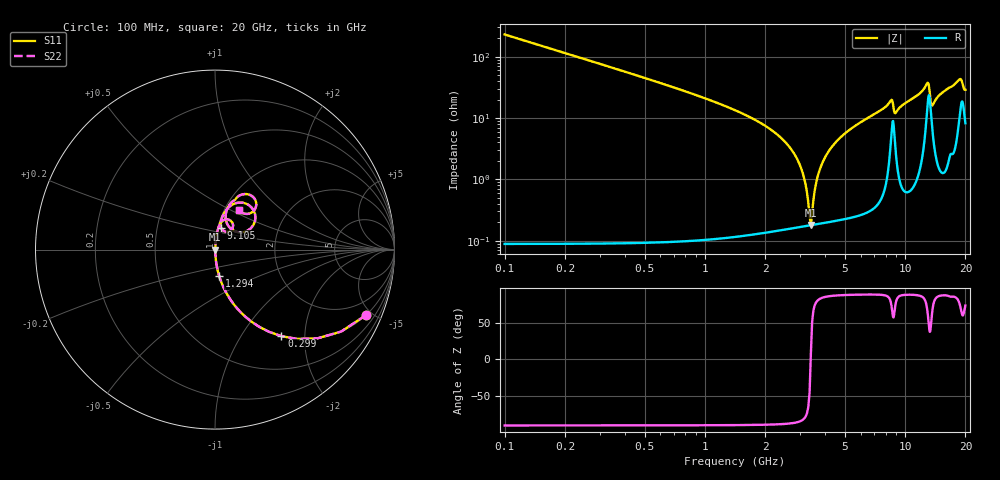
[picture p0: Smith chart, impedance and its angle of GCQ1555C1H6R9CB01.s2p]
!Murata Part Number: GCQ1555C1H6R9CB01
!These Parameters are Measured in Series Mode Connection
!Data Generated on Mar 13, 2026
!  o--ll--o
!Port1  Port2
!  o------o
!Operation Temp=25[degC], DC Bias Voltage=0[V]
!Freq. Start=100[MHz] Stop=20[GHz] 401[Steps]
# Hz S RI R 50
!Freq.(Hz) S11(Real) S11(Imag) S21(Real) S21(Imag) S12(Real) S12(Imag) S22(Real) S22(Imag)
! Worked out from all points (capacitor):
!   401 points, 100 MHz to 20 GHz, reference 50 ohm
!   read as one part in series: C = 6.9 pF near 199.5 MHz
!   lowest |Z| = 181 mohm at 3.384 GHz (marker M1)
!   series resonance near 3.378 GHz, so ESL is about 320 pH
!   S11 on the Smith chart (normalised r, x): 100 MHz: 1.00, -4.61; 299 MHz: 1.00, -1.53; 1.294 GHz: 1.00, -0.30; 9.105 GHz: 1.04, +0.26; 20 GHz: 1.16, +0.55
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1e8  0.8415 -0.3651  0.1585 0.3651  0.1585 0.3651  0.8415 -0.3651
2.99e8  0.3695 -0.4821  0.6305 0.4821  0.6305 0.4821  0.3695 -0.4821
5.975e8  0.1233 -0.3275  0.8767 0.3275  0.8767 0.3275  0.1233 -0.3275
1.294e9  0.0236 -0.1483  0.9764 0.1483  0.9764 0.1483  0.0236 -0.1483
2.7865e9  0.0023 -0.0264  0.9977 0.0264  0.9977 0.0264  0.0023 -0.0264
3.085e9  0.00185 -0.0124  0.9981 0.0124  0.9981 0.0124  0.00185 -0.0124
3.284e9  0.00177 -0.00384  0.9982 0.00384  0.9982 0.00384  0.00177 -0.00384
3.3835e9  0.00179 0.000238  0.9982 -0.000238  0.9982 -0.000238  0.00179 0.000238
3.43325e9  0.00181 0.00223  0.9982 -0.00223  0.9982 -0.00223  0.00181 0.00223
3.73175e9  0.00207 0.0137  0.9979 -0.0137  0.9979 -0.0137  0.00207 0.0137
4.279e9  0.00311 0.0327  0.9969 -0.0327  0.9969 -0.0327  0.00311 0.0327
6.7665e9  0.0145 0.1061  0.9855 -0.1061  0.9855 -0.1061  0.0145 0.1061
8.50775e9  0.0746 0.1676  0.9254 -0.1676  0.9254 -0.1676  0.0746 0.1676
8.856e9  0.0583 0.0999  0.9417 -0.0999  0.9417 -0.0999  0.0583 0.0999
9.10475e9  0.033 0.123  0.967 -0.123  0.967 -0.123  0.033 0.123
1.005e10  0.0357 0.1687  0.9643 -0.1687  0.9643 -0.1687  0.0357 0.1687
1.288575e10  0.1928 0.2446  0.8072 -0.2446  0.8072 -0.2446  0.1928 0.2446
1.338325e10  0.1429 0.0959  0.8571 -0.0959  0.8571 -0.0959  0.1429 0.0959
1.3632e10  0.0837 0.1207  0.9163 -0.1207  0.9163 -0.1207  0.0837 0.1207
1.67165e10  0.1078 0.2745  0.8922 -0.2745  0.8922 -0.2745  0.1078 0.2745
1.875625e10  0.2115 0.2938  0.7885 -0.2938  0.7885 -0.2938  0.2115 0.2938
2e10  0.1327 0.2214  0.8673 -0.2214  0.8673 -0.2214  0.1327 0.2214
